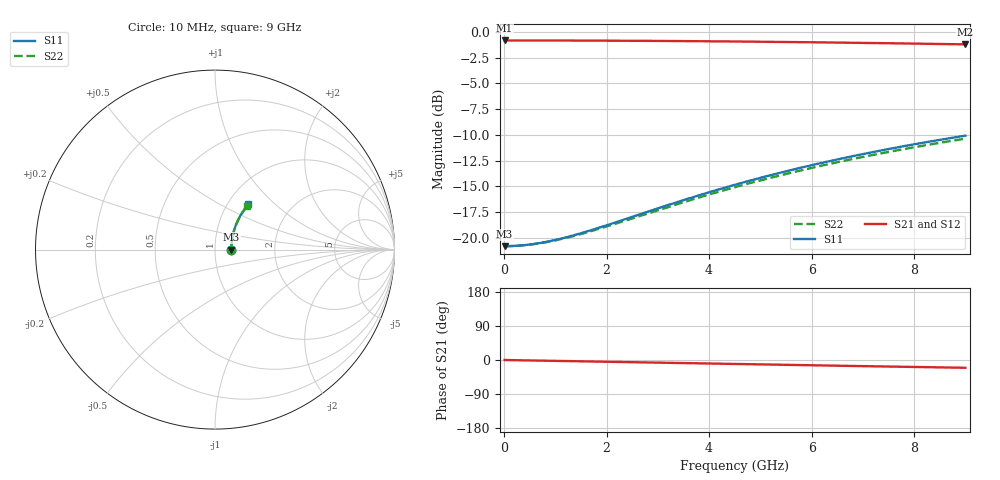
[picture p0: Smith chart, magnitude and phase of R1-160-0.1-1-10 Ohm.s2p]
!version-1
!date-03.2021
# MHz S RI R 50
!Freq ReS11 ImS11 ReS21 ImS21 ReS12 ImS12 ReS22 ImS22
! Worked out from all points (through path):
!   451 points, 10 MHz to 9 GHz, reference 50 ohm
!   highest |S21| = -0.83 dB at 10 MHz (marker M1); lowest = -1.2 dB at 9 GHz (marker M2)
!   group delay of S21, straight-line fit = 6.36 ps
!   lowest |S11| = -20.8 dB at 10 MHz (marker M3), VSWR 1.20, Z = 60 + j0.0383 ohm
!   |S11| at or under -10 dB: start of sweep to end of sweep
!   |S22| runs from -20.8 to -10.4 dB; largest |S21 - S12| = 0
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10  0.0909 0.000316  0.9091 -0.000374  0.9091 -0.000374  0.0909 0.000305
170  0.0909 0.00537  0.9091 -0.00636  0.9091 -0.00636  0.0909 0.00518
350  0.0911 0.0111  0.9089 -0.0131  0.9089 -0.0131  0.0911 0.0107
530  0.0913 0.0167  0.9087 -0.0198  0.9087 -0.0198  0.0913 0.0161
710  0.0916 0.0224  0.9084 -0.0265  0.9084 -0.0265  0.0915 0.0216
890  0.0919 0.0281  0.9081 -0.0333  0.9081 -0.0333  0.0919 0.0271
1090  0.0925 0.0344  0.9076 -0.0407  0.9076 -0.0407  0.0924 0.0331
1290  0.0931 0.0407  0.9069 -0.0481  0.9069 -0.0481  0.093 0.0392
1510  0.0939 0.0476  0.9061 -0.0563  0.9061 -0.0563  0.0937 0.0458
2030  0.0963 0.0638  0.9038 -0.0755  0.9038 -0.0755  0.096 0.0614
3010  0.1027 0.0938  0.8975 -0.1113  0.8975 -0.1113  0.1019 0.0904
3790  0.1094 0.1171  0.8909 -0.1392  0.8909 -0.1392  0.1082 0.1129
4150  0.113 0.1277  0.8873 -0.1519  0.8873 -0.1519  0.1116 0.1231
4510  0.1169 0.1381  0.8835 -0.1644  0.8835 -0.1644  0.1152 0.1332
4870  0.1211 0.1484  0.8794 -0.1768  0.8794 -0.1768  0.1192 0.1431
5250  0.1258 0.159  0.8747 -0.1897  0.8747 -0.1897  0.1236 0.1533
5630  0.1308 0.1694  0.8698 -0.2024  0.8698 -0.2024  0.1283 0.1634
6010  0.1361 0.1796  0.8645 -0.2149  0.8645 -0.2149  0.1332 0.1733
6750  0.1472 0.1989  0.8536 -0.2387  0.8536 -0.2387  0.1436 0.192
7510  0.1596 0.2177  0.8414 -0.2622  0.8414 -0.2622  0.1552 0.2103
8290  0.1732 0.236  0.8278 -0.2853  0.8278 -0.2853  0.168 0.2281
9000  0.1864 0.2517  0.8148 -0.3054  0.8148 -0.3054  0.1803 0.2433
